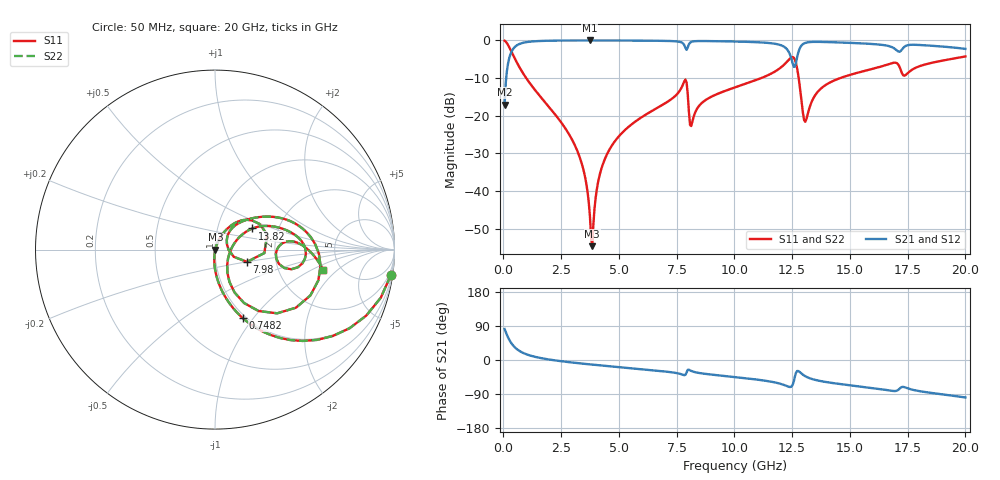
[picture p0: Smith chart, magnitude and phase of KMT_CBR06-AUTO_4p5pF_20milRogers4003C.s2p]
! Data measured by Modelithics Inc. support@modelithics.com 813-866-6335
! KEMET CBR06-AUTO 4.5pF, Pad Width= 0.851mm, Pad Length= 0.64mm, Pad Gap= 0.62mm, 20mil Rogers 4003C substrate Data, January 2022
# hz S ma R 50
! 2 Port Network Data from SP1.SP block
! freq  magS11  angS11  magS21  angS21  magS12  angS12  magS22  angS22
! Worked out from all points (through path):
!   401 points, 50 MHz to 20 GHz, reference 50 ohm
!   highest |S21| = -0.02 dB at 3.741 GHz (marker M1); lowest = -17.0 dB at 50 MHz (marker M2)
!   group delay of S21, straight-line fit = 15.5 ps
!   lowest |S11| = -54.6 dB at 3.841 GHz (marker M3), VSWR 1.00, Z = 50.2 + j0.0164 ohm
!   |S11| at or under -10 dB: 985.1 MHz to 11.16 GHz (10.18 GHz wide, 168 % of centre); 12.78 GHz to 14.58 GHz (1.798 GHz wide, 13.1 % of centre)
!   |S22| runs from -54.6 to -0.1 dB; largest |S21 - S12| = 0
!   S11 on the Smith chart (normalised r, x): 50 MHz: 1, -14; 748.2 MHz: 0.97, -0.89; 7.98 GHz: 1.42, -0.20; 13.82 GHz: 1.47, +0.37; 20 GHz: 3.67, -1.31
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5e7  0.99 -8.3  0.1411 81.7  0.1411 81.7  0.99 -8.3
2.99375e8  0.7585 -41.6  0.6508 48.4  0.6508 48.4  0.7585 -41.6
7.4825e8  0.4114 -67.9  0.9105 21.9  0.9105 21.9  0.4114 -67.9
3.391625e9  0.02312 -95.2  0.9979 -9.4  0.9979 -9.4  0.02312 -95.2
3.74075e9  0.00481 -80.1  0.9981 -11.5  0.9981 -11.5  0.00481 -80.1
3.8405e9  0.001863 5.0  0.9981 -12.1  0.9981 -12.1  0.001863 5.0
4.13975e9  0.01516 69.1  0.9979 -13.9  0.9979 -13.9  0.01516 69.1
4.588625e9  0.0356 70.4  0.9973 -16.5  0.9973 -16.5  0.0356 70.4
6.73325e9  0.1312 59.9  0.9879 -28.7  0.9879 -28.7  0.1312 59.9
7.8305e9  0.2867 29.8  0.8645 -40.2  0.8645 -40.2  0.2867 29.8
7.980125e9  0.191 -20.9  0.8093 -25.9  0.8093 -25.9  0.191 -20.9
8.179625e9  0.08364 38.2  0.9657 -30.1  0.9657 -30.1  0.08364 38.2
1.0025e10  0.2379 43.8  0.9661 -45.0  0.9661 -45.0  0.2379 43.8
1.202e10  0.4394 21.8  0.8612 -63.3  0.8612 -63.3  0.4394 21.8
1.251875e10  0.6008 -16.5  0.4992 -66.1  0.4992 -66.1  0.6008 -16.5
1.271825e10  0.4197 -54.6  0.6047 -28.9  0.6047 -28.9  0.4197 -54.6
1.30175e10  0.08775 -34.0  0.9124 -40.9  0.9124 -40.9  0.08775 -34.0
1.336662e10  0.1588 27.8  0.9546 -50.3  0.9546 -50.3  0.1588 27.8
1.38155e10  0.2394 29.4  0.9538 -56.6  0.9538 -56.6  0.2394 29.4
1.670825e10  0.4864 5.3  0.8368 -80.4  0.8368 -80.4  0.4864 5.3
1.74065e10  0.3453 0.1  0.8412 -72.7  0.8412 -72.7  0.3453 0.1
2e10  0.6127 -10.5  0.772 -98.8  0.772 -98.8  0.6127 -10.5
